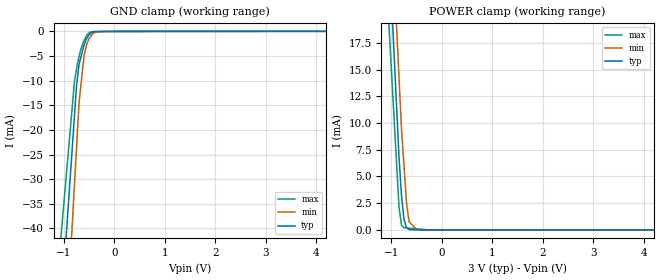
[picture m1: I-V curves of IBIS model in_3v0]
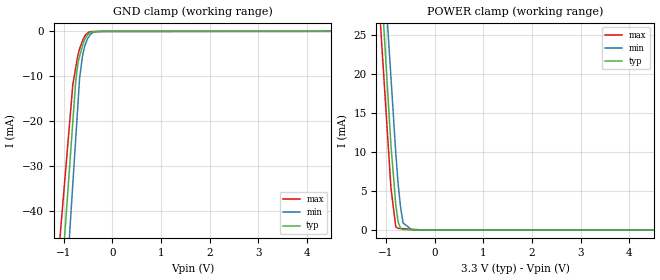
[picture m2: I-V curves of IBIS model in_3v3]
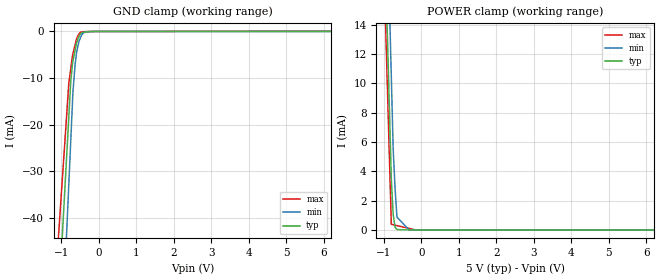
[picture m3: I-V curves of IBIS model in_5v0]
[IBIS Ver]   3.2
[Comment Char] |_char
[File Name]   tlv5639ipw.ibs
[File Rev]   3.0
[Source]
| This model file was created by Teraspeed Consulting Group LLC
| (http://www.teraspeed.com/).
[Date]   01-24-2008
[Notes]   Quality Check of this IBIS model: Model Passes IBIS Check
   Model parses into ICX IS. Simulation done with Hyperlynx.
   1. MIN TYP MAX information is based on Temprature and Voltage
   characteristics only.
[Disclaimer]
| This model is designed as an aid for customers of Texas Instruments.
| TI and its licensors and suppliers make no warranties, either expressed
| or implied, with respect to this  model, including the warranties of
| merchantability or fitness for a particular purpose.
| The model is provided solely on an "as is" basis. The entire risk as to
| its quality and performance is with the customer.
[Copyright]
| (C) Copyright 2008 Texas Instruments Incorporated. All rights reserved.
[Component] TLV5639IPW
[Manufacturer] TI
[Package]
| variable   typ   min   max
R_pkg  1.642E-02  1.490E-02  1.800E-02
L_pkg  2.070E-09  1.870E-09  2.270E-09
C_pkg  4.224E-13  3.820E-13  4.640E-13
[Pin] signal_name  model_name  R_pin  L_pin C_pin
1   D2   input  1.800E-02   2.270E-09   4.640E-13
2   D3   input  1.720E-02   2.170E-09   4.420E-13
3   D4   input  1.640E-02   2.070E-09   4.220E-13
4   D5   input  1.560E-02   1.970E-09   4.020E-13
5   D6   input  1.490E-02   1.870E-09   3.820E-13
6   D7   input  1.490E-02   1.870E-09   3.820E-13
7   D8   input  1.560E-02   1.970E-09   4.020E-13
8   D9   input  1.640E-02   2.070E-09   4.220E-13
9   D10   input  1.720E-02   2.170E-09   4.420E-13
10   D11   input  1.800E-02   2.270E-09   4.640E-13
11   VDD   POWER  1.800E-02   2.270E-09   4.640E-13
12   REF   analog 1.720E-02   2.170E-09   4.420E-13
13   OUT   analog 1.640E-02   2.070E-09   4.220E-13
14   AGND   GND   1.560E-02   1.970E-09   4.020E-13
15   REG   input  1.490E-02   1.870E-09   3.820E-13
16   _LDAC  input  1.490E-02   1.870E-09   3.820E-13
17   _WE   input  1.560E-02   1.970E-09   4.020E-13
18   _CS   input  1.640E-02   2.070E-09   4.220E-13
19   D0   input  1.720E-02   2.170E-09   4.420E-13
20   D1   input  1.800E-02   2.270E-09   4.640E-13
[Model Selector] input
in_3v0  3.0v input
in_3v3  3.3v input
in_5v0  5.0v input
[Model] analog
Model_type Terminator
C_comp  0pF 0pF 0pF
| variable typ   min   max
[Voltage Range]   5.00000V  4.50000V  5.50000V
[POWER Clamp Reference]  5.00000V  4.50000V  5.50000V
[GND Clamp Reference]   0.00000V  0.00000V  0.00000V
[Temperature Range]   25   85   -40
| Models and submodels in the file (4): in_3v0 (Input), in_3v3 (Input), in_5v0 (Input), analog (Terminator)
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[Model] in_3v0
Model_type Input
Vinl = 600.000mV
Vinh = 2.00000V
C_comp 916.00fF 916.00fF 916.00fF
| variable typ   min   max
[Voltage Range] 3.00000V 2.70000V 3.30000V
[POWER Clamp Reference] 3.00000V 2.70000V 3.30000V
[GND Clamp Reference] 0.00000V 0.00000V 0.00000V
[Temperature Range]   25   85   -40
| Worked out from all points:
|   GND clamp passes 1 mA (typ) near -0.52 V on its own axis
|   POWER clamp passes 1 mA (typ) near -0.75 V on its own axis
[GND Clamp]
-3V       -346.3mA   -437.7mA   -270.1mA
-790mV    -17.02mA   -31.02mA   -10.1mA
-750mV    -11.06mA   -23.66mA   -7.671mA
-730mV    -9.308mA   -19.98mA   -6.456mA
-700mV    -6.679mA   -14.46mA   -5.149mA
-670mV    -5.497mA   -11.57mA   -3.842mA
-600mV    -2.739mA   -4.835mA   -1.834mA
-550mV    -1.466mA   -2.71mA    -781.2uA
-490mV    -571.6uA   -1.304mA   -201.1uA
-400mV    -59.51uA   -261.7uA   -28.29uA
-175mV    -2.991uA   -5.192uA   -754.1nA
6V        5.183uA    22.51uA    72.88uA
[POWER Clamp]
-3V       219mA      225.1mA    198.2mA
-1.09V    30.55mA    37.83mA    22.63mA
-850mV    6.869mA    14.3mA     2.167mA
-800mV    3.213mA    9.402mA    453.4uA
-750mV    989.6uA    5.934mA    211.9uA
-700mV    222.6uA    2.467mA    190.9uA
-650mV    32.98uA    790.8uA    169.9uA
-500mV    17.76uA    21.06uA    107uA
-125mV    0A         0A         0A
6V        0A         0A         0A
[Model] in_3v3
Model_type Input
Vinl = 800.000mV
Vinh = 2.20000V
C_comp 916.00fF 916.00fF 916.00fF
| variable typ   min   max
[Voltage Range] 3.30000V 3.00000V 3.60000V
[POWER Clamp Reference] 3.30000V 3.00000V 3.60000V
[GND Clamp Reference] 0.00000V 0.00000V 0.00000V
[Temperature Range]   25   85   -40
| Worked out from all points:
|   GND clamp passes 1 mA (typ) near -0.52 V on its own axis
|   POWER clamp passes 1 mA (typ) near -0.75 V on its own axis
[GND Clamp]
-3.3V     -397.1mA   -454.1mA   -333.1mA
-810mV    -20.11mA   -33.95mA   -11.86mA
-750mV    -11.03mA   -23.82mA   -8.05mA
-700mV    -6.703mA   -15.38mA   -5.09mA
-670mV    -5.515mA   -10.32mA   -3.832mA
-610mV    -3.14mA    -5.429mA   -2.108mA
-570mV    -1.98mA    -3.437mA   -1.155mA
-490mV    -573.6uA   -1.347mA   -198.8uA
-450mV    -229.8uA   -688.8uA   -87.77uA
-390mV    -57.27uA   -213.8uA   -26.49uA
-165mV    -3.176uA   -3.407uA   -747nA
6.6V      5.785uA    10.82uA    74.84uA
[POWER Clamp]
-3.3V     258.3mA    253.3mA    242mA
-1.11V    32.53mA    40.02mA    25.85mA
-1.09V    30.47mA    38.07mA    23.88mA
-900mV    10.88mA    19.57mA    5.421mA
-800mV    3.239mA    9.828mA    379.9uA
-750mV    981.6uA    5.742mA    205.1uA
-700mV    185.1uA    2.833mA    184.8uA
-650mV    27.3uA     893.9uA    164.5uA
-470mV    12.18uA    20.8uA     91.38uA
-135mV    0A         0A         0A
6.6V      0A         0A         0A
[Model] in_5v0
Model_type Input
Vinl = 1.00000V
Vinh = 2.40000V
C_comp 916.00fF 916.00fF 916.00fF
| variable typ   min   max
[Voltage Range] 5.00000V 4.50000V 5.50000V
[POWER Clamp Reference] 5.00000V 4.50000V 5.50000V
[GND Clamp Reference] 0.00000V 0.00000V 0.00000V
[Temperature Range]   25   85   -40
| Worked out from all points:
|   GND clamp passes 1 mA (typ) near -0.52 V on its own axis
|   POWER clamp passes 1 mA (typ) near -0.75 V on its own axis
[GND Clamp]
-5V       -636.5mA   -788.1mA   -511.7mA
-800mV    -18.29mA   -32.75mA   -11.07mA
-750mV    -10.93mA   -23.76mA   -8.076mA
-700mV    -6.707mA   -14.77mA   -5.082mA
-690mV    -6.309mA   -12.97mA   -4.751mA
-630mV    -3.919mA   -6.889mA   -2.765mA
-590mV    -2.471mA   -4.358mA   -1.573mA
-530mV    -1.133mA   -2.158mA   -569.2uA
-450mV    -221.5uA   -718.7uA   -61.77uA
-330mV    -119.5uA   -48.86uA   -29.63uA
-165mV    -21.79uA   -3.385uA   -1.007uA
10V       2.477uA    4.615uA    83.19uA
[POWER Clamp]
-5V       395.6mA    425mA      412.9mA
-1.3V     50.14mA    59.78mA    45mA
-800mV    3.455mA    10.43mA    388uA
-750mV    1.045mA    5.493mA    358.1uA
-700mV    198.9uA    2.837mA    328.3uA
-650mV    29.2uA     881.9uA    298.4uA
-325mV    0A         0A         104.5uA
-110mV    0A         0A         0A
10V       0A         0A         0A
